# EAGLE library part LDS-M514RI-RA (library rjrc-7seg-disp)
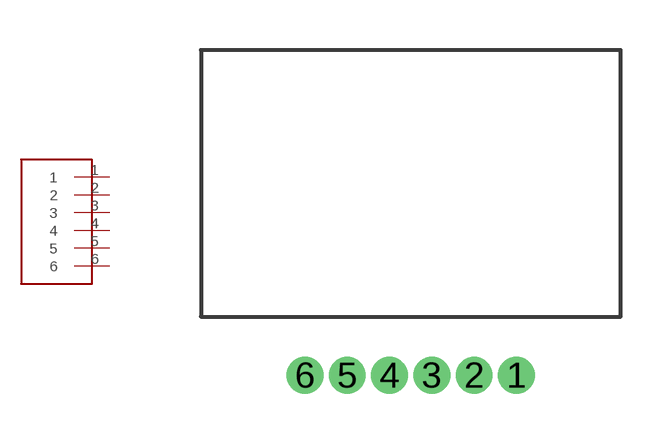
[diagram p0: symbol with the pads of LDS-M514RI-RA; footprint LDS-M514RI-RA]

Designator prefix -

## LDS-M514RI-RA  [LDS-M514RI-RA]
1  1
2  2
3  3
4  4
5  5
6  6

## Footprint LDS-M514RI-RA (pad centres in mm)
drill 0.6: 1 3.175,-5.753; 2 1.905,-5.753; 3 0.635,-5.753; 4 -0.635,-5.753; 5 -1.905,-5.753; 6 -3.175,-5.753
